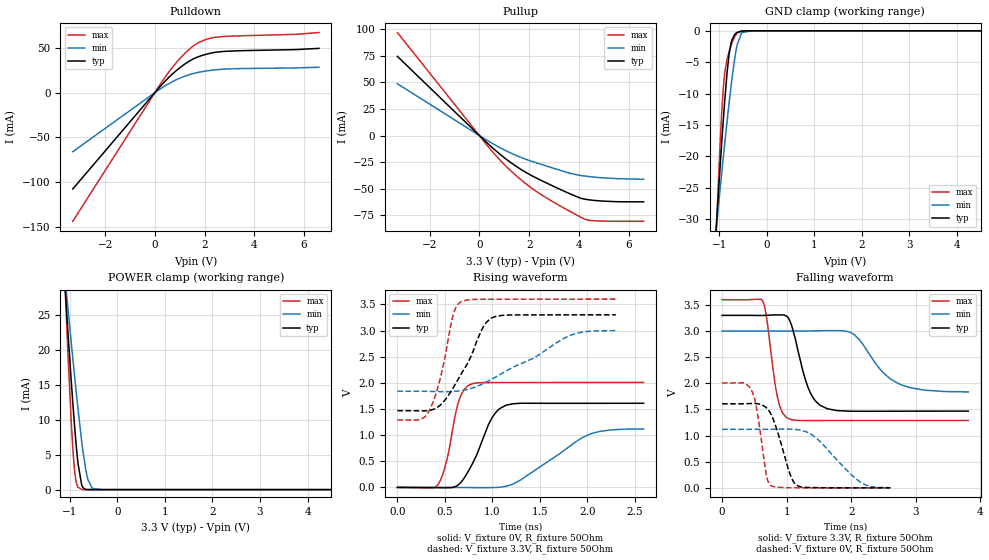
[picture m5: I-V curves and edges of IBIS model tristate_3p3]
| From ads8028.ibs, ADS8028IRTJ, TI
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|   tristate_3p3 Model
[Model]   tristate_3p3
Model_type   3-state
Polarity   Non-Inverting
Vmeas = 1.65
Vref = 0
Cref = 15pF
Rref = 150
|   typ   min   max
|   (nom PVT)   (fast PVT)   (slow PVT)
C_comp   1.258e-12   1.006e-12   1.516e-12
| Where nom  PVT is Nominal Process, 3.3V, 27C
|   Fast PVT is Strong Process,  3.6V, -40C
|   Slow PVT is Weak Process,   3V, 125C
[Voltage Range]   3.3   3   3.6
|Junction Temperature
[Temperature Range]   27   125   -40
[Pullup Reference]   3.3   3   3.6
[Pulldown Reference]   0   0   0
[Power Clamp Reference]   3.3   3   3.6
[GND Clamp Reference]   0   0   0
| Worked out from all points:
|   slope of the pulldown table from 0 to 0.495 V, typ, clamps not added: 32.5 ohm
|   slope of the pullup table from 0 to 0.495 V, typ, clamps not added: 45.4 ohm
|   GND clamp passes 1 mA (typ) near -0.70 V on its own axis
|   POWER clamp passes 1 mA (typ) near -0.76 V on its own axis
|   falling waveform, V_fixture 3.3V, R_fixture 50Ohm: 20-80 % time 246ps typ, 464ps min, 152ps max; typ from 3.3 V to 1.47 V
|   rising waveform, V_fixture 0V, R_fixture 50Ohm: 20-80 % time 233ps typ, 534ps min, 136ps max; typ from 0 V to 1.61 V
|   rising waveform, V_fixture 3.3V, R_fixture 50Ohm: 20-80 % time 305ps typ, 680ps min, 168ps max; typ from 1.47 V to 3.3 V
|   falling waveform, V_fixture 0V, R_fixture 50Ohm: 20-80 % time 236ps typ, 515ps min, 144ps max; typ from 1.61 V to 0 V
[Pulldown]
|   Voltage   I(typ)   I(min)   I(max)
-3.3V     -107.8mA   -66.09mA   -144mA
276mV     8.84mA     5.278mA    11.96mA
580.8mV   17.61mA    10.41mA    23.89mA
922.8mV   26.13mA    15.26mA    35.64mA
1.254V    33.01mA    18.98mA    45.31mA
1.582V    38.28mA    21.68mA    53.01mA
2.043V    42.88mA    24.23mA    59.41mA
2.439V    45.28mA    25.69mA    62.1mA
3.231V    46.84mA    26.88mA    63.5mA
5.683V    48.3mA     27.77mA    65.41mA
6.6V      49.64mA    28.48mA    67.35mA
[GND Clamp]
|   Voltage   I(typ)   I(min)   I(max)
-3.3V     -329.5mA   -221.2mA   -503mA
-1.069V   -31.97mA   -31.97mA   -33.26mA
-1.007V   -24.53mA   -27.12mA   -22.09mA
-947.1mV  -17.71mA   -22.57mA   -12.88mA
-918mV    -14.56mA   -20.39mA   -9.418mA
-884.4mV  -11.11mA   -17.92mA   -6.677mA
-792mV    -3.682mA   -11.43mA   -3.306mA
-749.1mV  -1.863mA   -8.65mA    -2.279mA
-623.7mV  -249.1uA   -2.22mA    -381.1uA
-528mV    -34.24uA   -305.9uA   -38.64uA
-330mV    -163.9nA   -2.067uA   -60.66nA
6.6V      0A         0A         0A
[Pullup]
|   Voltage   I(typ)   I(min)   I(max)
-3.3V     74.5mA     48.76mA    96.9mA
459mV     -10.15mA   -6.561mA   -13.4mA
1.137V    -23.27mA   -15.06mA   -30.34mA
1.981V    -36.14mA   -23.22mA   -47.38mA
2.946V    -47.34mA   -30.46mA   -62.15mA
3.633V    -54.7mA    -35.42mA   -71.21mA
4.069V    -58.91mA   -37.5mA    -76.67mA
4.245V    -59.81mA   -38.09mA   -78.71mA
4.788V    -61.31mA   -39.42mA   -80.27mA
6.6V      -62.28mA   -41.06mA   -80.59mA
[POWER Clamp]
|   Voltage   I(typ)   I(min)   I(max)
-3.3V     266.8mA    193.9mA    379.8mA
-1.158V   35.09mA    34.37mA    37.89mA
-1.054V   23.71mA    26.73mA    21.21mA
-970.8mV  15.33mA    20.89mA    9.481mA
-938.4mV  12.28mA    18.66mA    5.771mA
-904.2mV  9.237mA    16.34mA    2.838mA
-877.2mV  7.016mA    14.54mA    1.388mA
-831.6mV  3.796mA    11.6mA     344.4uA
-752.4mV  634.8uA    6.865mA    24.22uA
-624mV    6.907uA    1.455mA    326.4nA
-531mV    249.5nA    180.1uA    12.48nA
6.6V      0A         0A         0A
[Ramp]
R_load = 50
|   typ   min   max
dV/dt_r   0.96517/2.31784e-10   0.672063/5.32464e-10   1.20373/1.3583e-10
dV/dt_f   1.09944/2.44212e-10   0.696857/4.54774e-10   1.38667/1.51444e-10
[Falling Waveform]
V_fixture = 3.3V
V_fixture_min = 3V
V_fixture_max = 3.6V
R_fixture = 50Ohm
|   Time   V(typ)   V(min)   V(max)
0s        3.3V       3V         3.6V
624ps     3.298V     3V         3.583V
688ps     3.301V     3V         3.268V
852ps     3.309V     3V         1.768V
1.006ns   3.277V     3V         1.339V
1.33ns    1.926V     3.001V     1.287V
1.522ns   1.577V     3.006V     1.288V
2.012ns   1.466V     2.958V     1.289V
2.798ns   1.467V     1.961V     1.289V
3.812ns   1.468V     1.835V     1.289V
[Rising Waveform]
V_fixture = 0V
V_fixture_min = 0V
V_fixture_max = 0V
R_fixture = 50Ohm
|   Time   V(typ)   V(min)   V(max)
0s        1.753nV    11.11nV    1.447nV
428ps     -5.203mV   285.1uV    56.78mV
518ps     -5.75mV    -86.85uV   507.3mV
642ps     51.87mV    -1.241mV   1.627V
698ps     166.3mV    -1.96mV    1.859V
760ps     352.3mV    -2.829mV   1.961V
994ps     1.325V     -2.958mV   2.005V
1.142ns   1.569V     21.32mV    2.005V
2.006ns   1.608V     1.004V     2.007V
2.592ns   1.609V     1.119V     2.007V
[Rising Waveform]
V_fixture = 3.3V
V_fixture_min = 3V
V_fixture_max = 3.6V
R_fixture = 50Ohm
|   Time   V(typ)   V(min)   V(max)
0s        1.468V     1.839V     1.289V
224ps     1.464V     1.839V     1.293V
348ps     1.477V     1.836V     1.511V
452ps     1.575V     1.832V     2.093V
590ps     1.913V     1.835V     3.318V
672ps     2.171V     1.85V      3.551V
906ps     3.077V     1.987V     3.597V
990ps     3.24V      2.065V     3.598V
1.824ns   3.299V     2.91V      3.6V
2.3ns     3.3V       3V         3.6V
[Falling Waveform]
V_fixture = 0V
V_fixture_min = 0V
V_fixture_max = 0V
R_fixture = 50Ohm
|   Time   V(typ)   V(min)   V(max)
0s        1.608V     1.12V      2.005V
470ps     1.614V     1.12V      1.832V
544ps     1.609V     1.12V      1.453V
680ps     1.54V      1.121V     278mV
748ps     1.431V     1.122V     50.65mV
1.048ns   279.4mV    1.123V     2.292mV
1.154ns   50.79mV    1.115V     1.039mV
1.492ns   3.736mV    917.2mV    444.7uV
2.138ns   348.4uV    112.7mV    166.7uV
2.606ns   186.2uV    4.19mV     69.34uV
